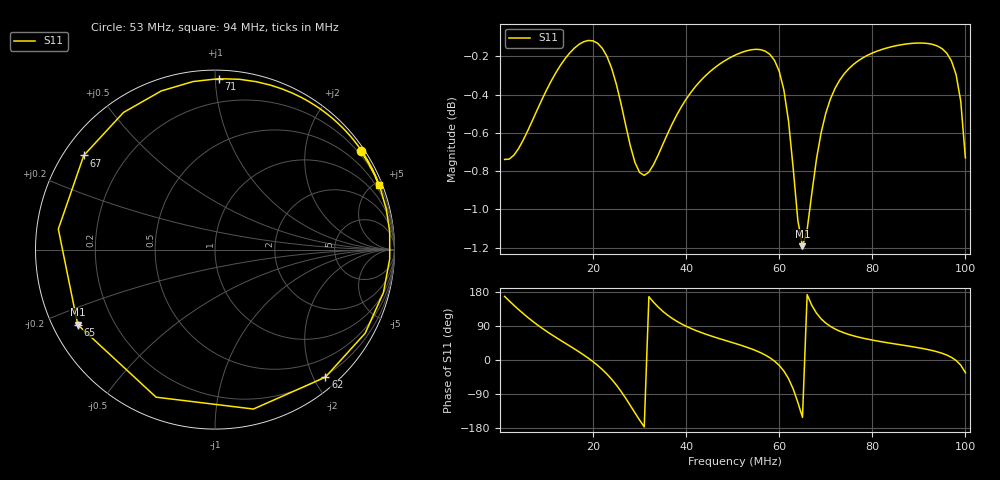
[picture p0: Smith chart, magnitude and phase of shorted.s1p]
# MHz S RI R 50.0
! SimSmith 18.4f
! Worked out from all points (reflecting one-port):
!   100 points, 1 MHz to 100 MHz, reference 50 ohm
!   lowest |S11| = -1.2 dB at 65 MHz (marker M1), VSWR 14.59, Z = 3.65 - j12.7 ohm
!   phase of S11 starts at 168 deg and turns -921 deg over the sweep
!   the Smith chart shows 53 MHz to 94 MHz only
!   S11 on the Smith chart (normalised r, x): 53 MHz: 0.12, +3.28; 62 MHz: 0.18, -2.17; 65 MHz: 0.07, -0.25; 67 MHz: 0.06, +0.32; 71 MHz: 0.05, +1.02; 94 MHz: 0.24, +5.27
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1  -0.8976 0.1944
4  -0.6322 0.6745
7  -0.2019 0.9185
14  0.6964 0.6837
18  0.9596 0.2264
21  0.9542 -0.2444
24  0.6131 -0.752
26  0.1238 -0.9418
28  -0.4606 -0.8035
31  -0.908 -0.0554
35  -0.575 0.7269
39  -0.0871 0.9441
51  0.7281 0.6538
53  0.814 0.5467
59  0.9735 -0.0517
62  0.6148 -0.7109
63  0.2142 -0.8882
64  -0.3282 -0.8223
65  -0.7647 -0.4184
66  -0.8729 0.1145
67  -0.731 0.5246
69  -0.2993 0.884
71  0.0208 0.9523
76  0.4315 0.8717
88  0.7935 0.5833
94  0.9152 0.3596
98  0.9664 -0.0209
100  0.7671 -0.5067
